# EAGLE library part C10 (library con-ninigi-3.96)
NINIGI
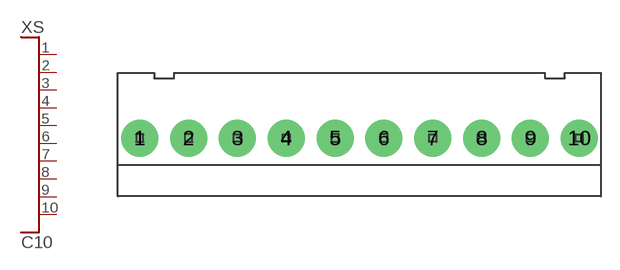
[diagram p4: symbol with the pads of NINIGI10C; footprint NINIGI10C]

Designator prefix XS

## C10  [NINIGI10C]
1  P$1
2  P$2
3  P$3
4  P$4
5  P$5
6  P$6
7  P$7
8  P$8
9  P$9
10  P$10

## Footprint NINIGI10C (pad centres in mm)
drill 1.6 pad 3: 1 -17.82,0; 2 -13.86,0; 3 -9.9,0; 4 -5.94,0; 5 -1.98,0; 6 1.98,0; 7 5.94,0; 8 9.9,0; 9 13.86,0; 10 17.82,0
